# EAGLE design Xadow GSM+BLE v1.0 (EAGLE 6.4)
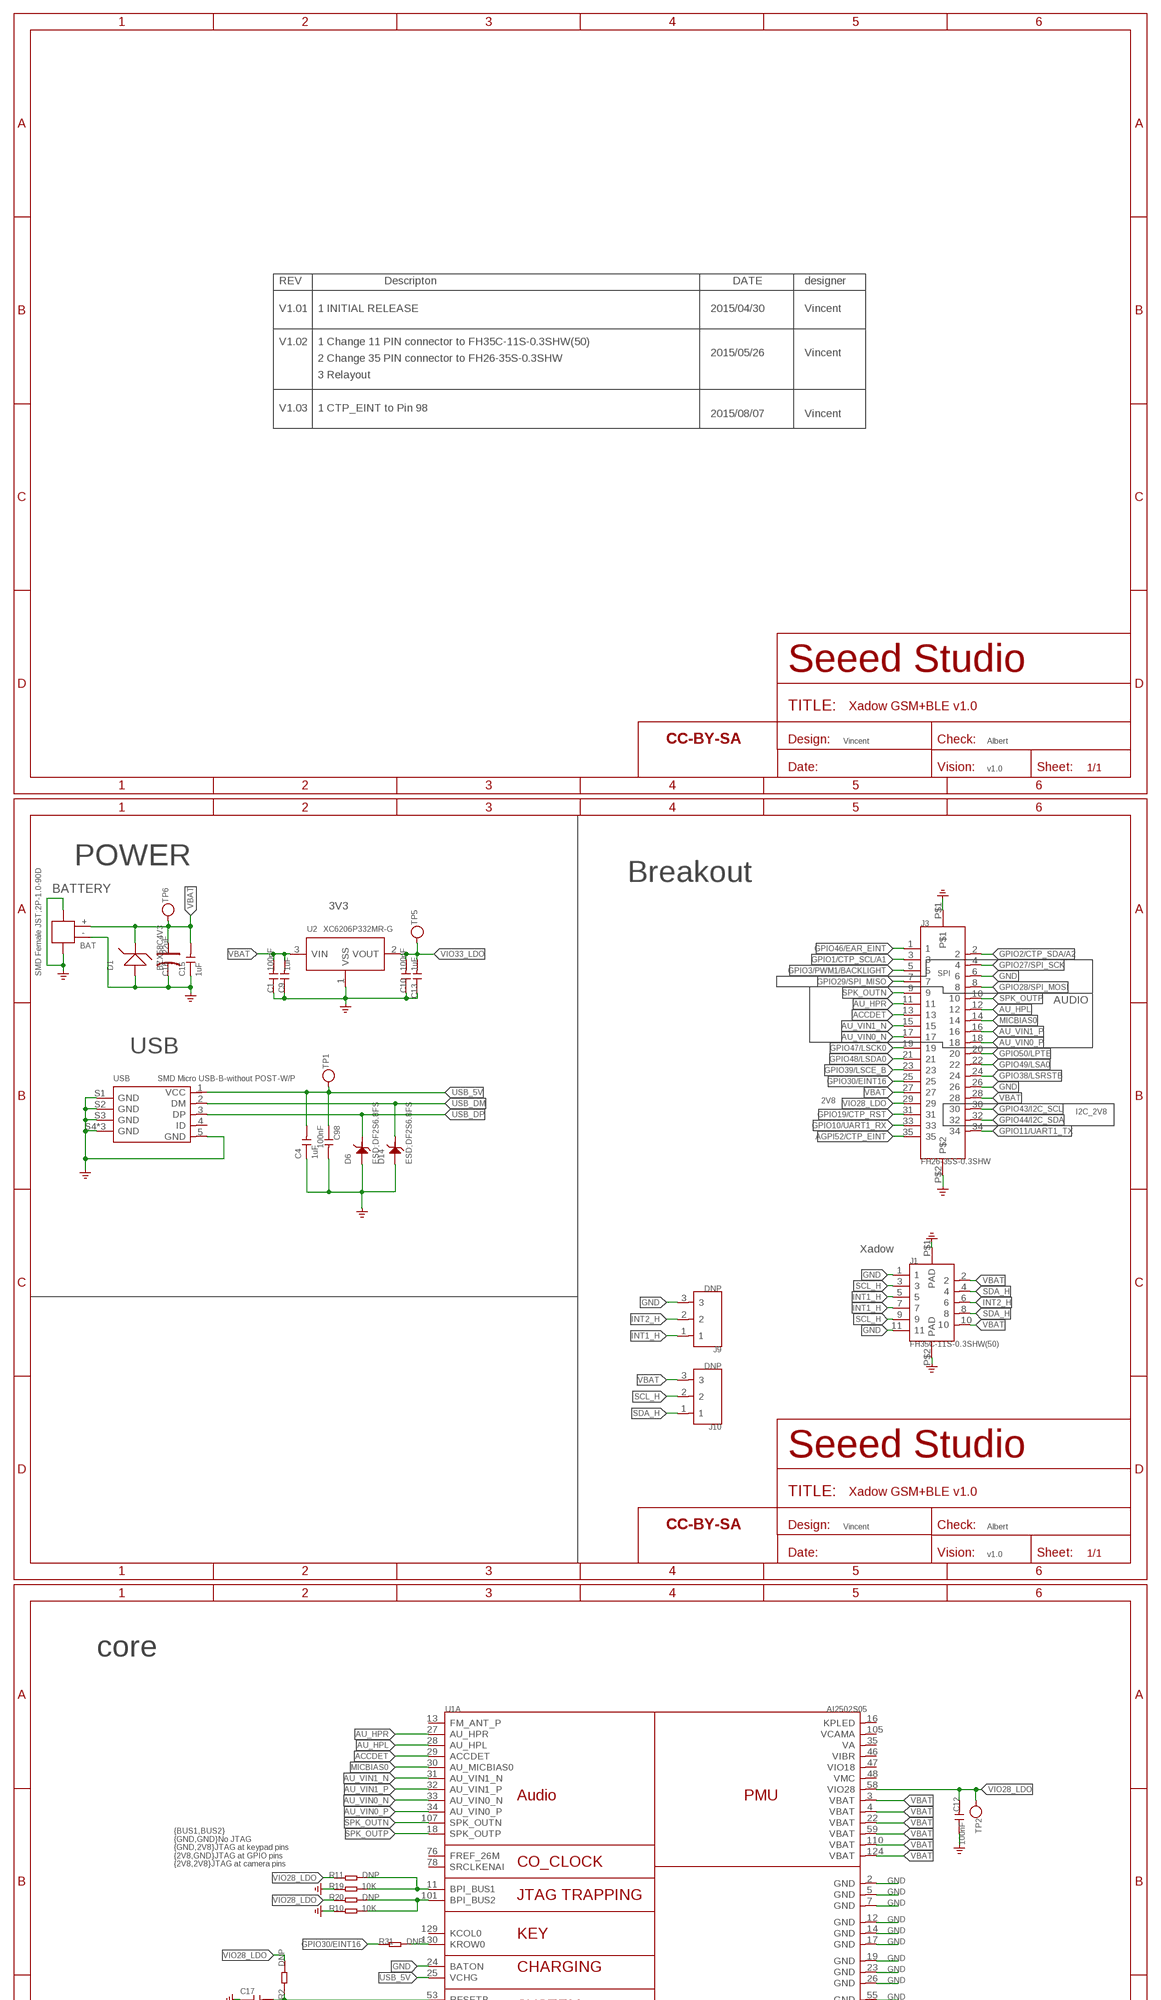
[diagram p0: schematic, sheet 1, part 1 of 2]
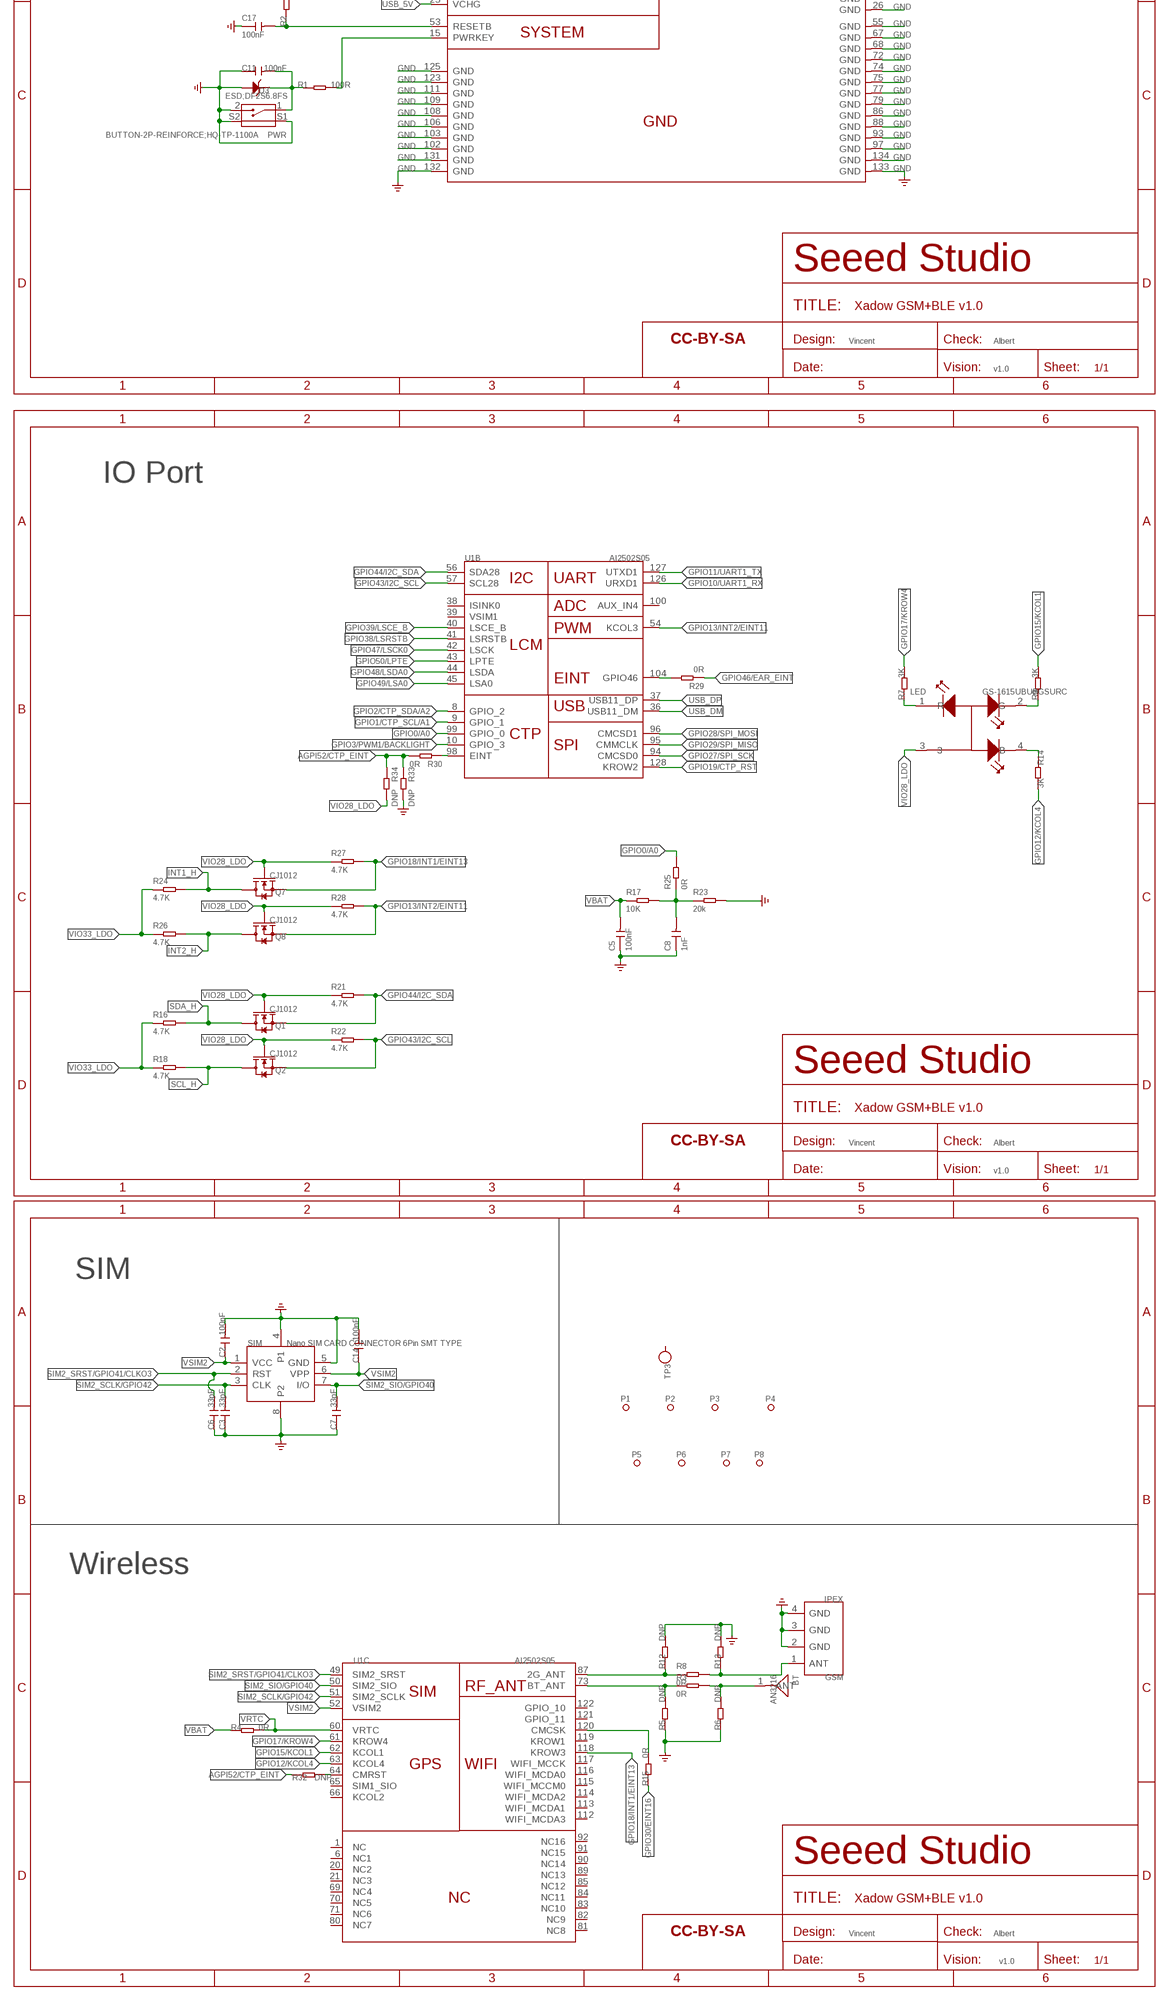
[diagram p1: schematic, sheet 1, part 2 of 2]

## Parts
BAT  SMD Female JST;2P-1.0-90D  JST-2P-SMD'1.0'  [HW2-SMD-1.0-90D]
BT  AN3216  ANTENNA-AN3216  [ANT-SMD2P-3.2X1.6X1.04MM]
C1  100nF  CAP-0201  [C0201]
C2  100nF  CAP-0201  [C0201]
C3  33pF  CAP-0201  [C0201]
C4  1uF  CAP-0402  [C0402]
C5  100nF  CAP-0201  [C0201]
C6  33pF  CAP-0201  [C0201]
C7  33pF  CAP-0201  [C0201]
C8  1nF  CAP-0201  [C0201]
C9  1uF  CAP-0402  [C0402]
C10  100nF  CAP-0201  [C0201]
C11  100nF  CAP-0201  [C0201]
C12  100nF  CAP-0201  [C0201]
C13  1uF  CAP-0402  [C0402]
C14  100nF  CAP-0201  [C0201]
C15  1uF  CAP-0402  [C0402]
C16  22uF  CAP-POLAR-AVX-A  [AVX-A]
C17  100nF  CAP-0201  [C0201]
C98  100nF  CAP-0201  [C0201]
D1  BZX58C4V3  D-ZENER-2P'BZX584CX'  [SOD-523]
D3  ESD;DF2S6.8FS  D-ESD-2P'DF2S6.8FS'  [SOD-923]
D6  ESD;DF2S6.8FS  D-ESD-2P'DF2S6.8FS'  [SOD-923]
D14  ESD;DF2S6.8FS  D-ESD-2P'DF2S6.8FS'  [SOD-923]
FR1  SEEEDSTUDIO-OPEN-SCH-FRAME  [SEEEDSTUDIO-PCB-FRAME]
GSM  IPEX  ANT_IPEX  [ANT-IPEX4-1.7X1.7MM]
J1  FH35C-11S-0.3SHW(50)  FPC-CONNECTER-11P(FH35C-11S-0.3SHW(50))  [FPC11-SMD-0.3(FH35C)]
J3  FH26-35S-0.3SHW  FPC-CONNECTER-35P(FH26W-35S-0.3SHW(10))  [FPC35-SMD-0.3(FH26W)]
J9  DNP  HEADER3  [3P-DIP-2]
J10  DNP  HEADER3  [3P-DIP-2]
LED  GS-1615UBUBGSURC  LED-GS-0603RGB  [LED-SMD4P-1.6X1.5MM]
P1  MARK-1.0'ANNULAR'  [ROUND-MARK-1.0]
P2  MARK-1.0'ANNULAR'  [ROUND-MARK-1.0]
P3  MARK-1.0'ANNULAR'  [ROUND-MARK-1.0]
P4  MARK-1.0'ANNULAR'  [ROUND-MARK-1.0]
P5  MARK-1.0'ANNULAR'  [ROUND-MARK-1.0]
P6  MARK-1.0'ANNULAR'  [ROUND-MARK-1.0]
P7  MARK-1.0'ANNULAR'  [ROUND-MARK-1.0]
P8  MARK-1.0'ANNULAR'  [ROUND-MARK-1.0]
PWR  BUTTON-2P-REINFORCE;HQ-TP-1100A  BUTTON-2+2P'HQ-TP-1100A'  [SW4-SMD-4.5X3.8X1.8MM-90D]
Q1  CJ1012  MOSFET-N  [SOT-523]
Q2  CJ1012  MOSFET-N  [SOT-523]
Q7  CJ1012  MOSFET-N  [SOT-523]
Q8  CJ1012  MOSFET-N  [SOT-523]
R1  100R  RES-0201  [R0201]
R2  DNP  RES-0201  [R0201]
R3  0R  RES-0201  [R0201]
R4  0R  RES-0201  [R0201]
R5  DNP  RES-0201  [R0201]
R6  DNP  RES-0201  [R0201]
R7  3K  RES-0201  [R0201]
R8  0R  RES-0201  [R0201]
R9  3K  RES-0201  [R0201]
R10  10K  RES-0201  [R0201]
R11  DNP  RES-0201  [R0201]
R12  DNP  RES-0201  [R0201]
R13  DNP  RES-0201  [R0201]
R14  3K  RES-0201  [R0201]
R15  0R  RES-0201  [R0201]
R16  4.7K  RES-0201  [R0201]
R17  10K  RES-0201  [R0201]
R18  4.7K  RES-0201  [R0201]
R19  10K  RES-0201  [R0201]
R20  DNP  RES-0201  [R0201]
R21  4.7K  RES-0201  [R0201]
R22  4.7K  RES-0201  [R0201]
R23  20k  RES-0201  [R0201]
R24  4.7K  RES-0201  [R0201]
R25  0R  RES-0201  [R0201]
R26  4.7K  RES-0201  [R0201]
R27  4.7K  RES-0201  [R0201]
R28  4.7K  RES-0201  [R0201]
R29  0R  RES-0201  [R0201]
R30  0R  RES-0201  [R0201]
R31  DNP  RES-0201  [R0201]
R32  DNP  RES-0201  [R0201]
R33  DNP  RES-0201  [R0201]
R34  DNP  RES-0201  [R0201]
SIM  Nano SIM CARD CONNECTOR 6Pin SMT TYPE  NANO-SIM-6+2P-SMD  [NANO-SIM6+2P-SMD-12.3X10X1.5MM]
TP1  PAD-TEST-POINT  [TP-D23MIL]
TP2  PAD-TEST-POINT  [TP-D23MIL]
TP3  PAD-TEST-POINT  [TP-D23MIL]
TP5  PAD-TEST-POINT  [TP-D23MIL]
TP6  PAD-TEST-POINT  [TP-D23MIL]
U1  AI2502S05  MODULE-MT2502A  [LGA134-0.6-17X15MM]
U2  XC6206P332MR-G  PMIC-XC6206PMR  [SOT-23]
U$1  SEEEDSTUDIO-OPEN-SCH-FRAME  [SEEEDSTUDIO-PCB-FRAME]
U$3  SEEEDSTUDIO-OPEN-SCH-FRAME  [SEEEDSTUDIO-PCB-FRAME]
U$5  SEEEDSTUDIO-OPEN-SCH-FRAME  [SEEEDSTUDIO-PCB-FRAME]
U$11  SEEEDSTUDIO-OPEN-SCH-FRAME  [SEEEDSTUDIO-PCB-FRAME]
USB  SMD Micro USB-B-without POST-W/P  MICRO-USB5+4P  [MICRO-USB5+4P-SMD-0.65-B-NO-HOLE]

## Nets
ACCDET: J3.13 U1.29(A:ACCDET)
AGPI52/CTP_EINT: J3.35 R30.2 R32.1 R33.1 R34.1
AU_HPL: J3.12 U1.28(A:AU_HPL)
AU_HPR: J3.11 U1.27(A:AU_HPR)
AU_VIN0_N: J3.17 U1.33(A:AU_VIN0_N)
AU_VIN0_P: J3.18 U1.34(A:AU_VIN0_P)
AU_VIN1_N: J3.15 U1.31(A:AU_VIN1_N)
AU_VIN1_P: J3.16 U1.32(A:AU_VIN1_P)
GND: BAT.3 BAT.4 BAT.- C1.1 C2.2 C3.1 C4.1 C5.1 C6.1 C7.1 C8.1 C9.1 C10.1 C11.1 C12.1 C13.1 C14.2 C15.1 C16.- C17.1 C98.2 D1.+ D3.2 D6.2 D14.2 GSM.2(GND) GSM.3(GND) GSM.4(GND) J1.1 J1.11 J1.P$1(PAD) J1.P$2(PAD) J3.6 J3.26 J3.P$1 J3.P$2 J9.3 PWR.2 PWR.S1 PWR.S2 R5.1 R6.1 R10.1 R12.2 R13.2 R19.1 R23.2 R33.2 SIM.4(P1) SIM.5(GND) SIM.8(P2) U1.2(A:GND) U1.5(A:GND) U1.7(A:GND) U1.12(A:GND) U1.14(A:GND) U1.17(A:GND) U1.19(A:GND) U1.23(A:GND) U1.24(A:BATON) U1.26(A:GND) U1.55(A:GND) U1.67(A:GND) U1.68(A:GND) U1.72(A:GND) U1.74(A:GND) U1.75(A:GND) U1.77(A:GND) U1.79(A:GND) U1.86(A:GND) U1.88(A:GND) U1.93(A:GND) U1.97(A:GND) U1.102(A:GND) U1.103(A:GND) U1.106(A:GND) U1.108(A:GND) U1.109(A:GND) U1.111(A:GND) U1.123(A:GND) U1.125(A:GND) U1.131(A:GND) U1.132(A:GND) U1.133(A:GND) U1.134(A:GND) U2.1(VSS) USB.5(GND) USB.S1(GND) USB.S2(GND) USB.S3(GND) USB.S4(GND) USB.S5(GND) USB.S6(GND) ; supply symbol labelled GND_POWER
GPIO0/A0: R25.2 U1.99(B:GPIO_0)
GPIO1/CTP_SCL/A1: J3.3 U1.9(B:GPIO_1)
GPIO2/CTP_SDA/A2: J3.2 U1.8(B:GPIO_2)
GPIO3/PWM1/BACKLIGHT: J3.5 U1.10(B:GPIO_3)
GPIO10/UART1_RX: J3.33 U1.126(B:URXD1)
GPIO11/UART1_TX: J3.34 U1.127(B:UTXD1)
GPIO12/KCOL4: R14.2 U1.63(C:KCOL4)
GPIO13/INT2/EINT11: Q8.2(S) R28.2 U1.54(B:KCOL3)
GPIO15/KCOL1: R9.2 U1.62(C:KCOL1)
GPIO17/KROW4: R7.2 U1.61(C:KROW4)
GPIO18/INT1/EINT13: Q7.2(S) R27.2 U1.118(C:KROW3)
GPIO19/CTP_RST: J3.31 U1.128(B:KROW2)
GPIO27/SPI_SCK: J3.4 U1.94(B:CMCSD0)
GPIO28/SPI_MOSI: J3.8 U1.96(B:CMCSD1)
GPIO29/SPI_MISO: J3.7 U1.95(B:CMMCLK)
GPIO30/EINT16: J3.25 R15.1 R31.1
GPIO38/LSRSTB: J3.24 U1.41(B:LSRSTB)
GPIO39/LSCE_B: J3.23 U1.40(B:LSCE_B)
GPIO43/I2C_SCL: J3.30 Q2.2(S) R22.2 U1.57(B:SCL28)
GPIO44/I2C_SDA: J3.32 Q1.2(S) R21.2 U1.56(B:SDA28)
GPIO46/EAR_EINT: J3.1 R29.1
GPIO47/LSCK0: J3.19 U1.42(B:LSCK)
GPIO48/LSDA0: J3.21 U1.44(B:LSDA)
GPIO49/LSA0: J3.22 U1.45(B:LSA0)
GPIO50/LPTE: J3.20 U1.43(B:LPTE)
INT1_H: J1.5 J1.7 J9.1 Q7.3(D) R24.2
INT2_H: J1.6 J9.2 Q8.3(D) R26.2
MICBIAS0: J3.14 U1.30(A:AU_MICBIAS0)
N$1: R15.2 U1.120(C:CMCSK)
N$2: R29.2 U1.104(B:GPIO46)
N$3: R30.1 U1.98(B:EINT)
N$4: BT.1(ANT) R3.2 R6.2
N$5: R8.1 R12.1 U1.87(C:2G_ANT)
N$6: R31.2 U1.130(A:KROW0)
N$7: GSM.1(ANT) R8.2 R13.1
N$8: C11.2 D3.1 PWR.1 R1.1
N$9: R3.1 R5.2 U1.73(C:BT_ANT)
N$10: R1.2 U1.15(A:PWRKEY)
N$12: C8.2 R17.2 R23.1 R25.1
N$18: R32.2 U1.64(C:CMRST)
N$20: R10.2 R20.2 U1.101(A:BPI_BUS2)
N$21: R11.2 R19.2 U1.11(A:BPI_BUS1)
N$32: LED.1(R) R7.1
N$33: LED.2(G) R9.1
N$34: LED.4(B) R14.1
RESETB: C17.2 R2.1 U1.53(A:RESETB)
SCL_H: J1.3 J1.9 J10.2 Q2.3(D) R18.2
SDA_H: J1.4 J1.8 J10.1 Q1.3(D) R16.2
SIM2_SCLK/GPIO42: C3.2 SIM.3(CLK) U1.51(C:SIM2_SCLK)
SIM2_SIO/GPIO40: C7.2 SIM.7(I/O) U1.50(C:SIM2_SIO)
SIM2_SRST/GPIO41/CLKO3: C6.2 SIM.2(RST) U1.49(C:SIM2_SRST)
SPK_OUTN: J3.9 U1.107(A:SPK_OUTN)
SPK_OUTP: J3.10 U1.18(A:SPK_OUTP)
USB_5V: C4.2 C98.1 TP1.T U1.25(A:VCHG) USB.1(VCC)
USB_DM: D14.1 U1.36(B:USB11_DM) USB.2(DM)
USB_DP: D6.1 U1.37(B:USB11_DP) USB.3(DP)
VBAT: BAT.+ C1.2 C5.2 C9.2 C15.2 C16.+ D1.- J1.2 J1.10 J3.27 J3.28 J10.3 R4.1 R17.1 TP6.T U1.3(A:VBAT) U1.4(A:VBAT) U1.22(A:VBAT) U1.59(A:VBAT) U1.110(A:VBAT) U1.124(A:VBAT) U2.3(VIN)
VIO28_LDO: C12.2 J3.29 LED.3 Q1.1(G) Q2.1(G) Q7.1(G) Q8.1(G) R2.2 R11.1 R20.1 R21.1 R22.1 R27.1 R28.1 R34.2 TP2.T U1.58(A:VIO28)
VIO33_LDO: C10.2 C13.2 R16.1 R18.1 R24.1 R26.1 TP5.T U2.2(VOUT)
VRTC: R4.2 U1.60(C:VRTC)
VSIM2: C2.1 C14.1 SIM.1(VCC) SIM.6(VPP) U1.52(C:VSIM2)
Unconnected: TP3.T U1.1(C:NC) U1.6(C:NC1) U1.13(A:FM_ANT_P) U1.16(A:KPLED) U1.20(C:NC2) U1.21(C:NC3) U1.35(A:VA) U1.38(B:ISINK0) U1.39(B:VSIM1) U1.46(A:VIBR) U1.47(A:VIO18) U1.48(A:VMC) U1.65(C:SIM1_SIO) U1.66(C:KCOL2) U1.69(C:NC4) U1.70(C:NC5) U1.71(C:NC6) U1.76(A:FREF_26M) U1.78(A:SRCLKENAI) U1.80(C:NC7) U1.81(C:NC8) U1.82(C:NC9) U1.83(C:NC10) U1.84(C:NC11) U1.85(C:NC12) U1.89(C:NC13) U1.90(C:NC14) U1.91(C:NC15) U1.92(C:NC16) U1.100(B:AUX_IN4) U1.105(A:VCAMA) U1.112(C:WIFI_MCDA3) U1.113(C:WIFI_MCDA1) U1.114(C:WIFI_MCDA2) U1.115(C:WIFI_MCCM0) U1.116(C:WIFI_MCDA0) U1.117(C:WIFI_MCCK) U1.119(C:KROW1) U1.121(C:GPIO_11) U1.122(C:GPIO_10) U1.129(A:KCOL0) USB.4(ID)

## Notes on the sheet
- REV | Descripton | DATE | designer
- V1.01 | 1 INITIAL RELEASE | 2015/04/30 | Vincent
- V1.02 | 1 Change 11 PIN connector to FH35C-11S-0.3SHW(50)
- 2015/05/26 | Vincent
- 2 Change 35 PIN connector to FH26-35S-0.3SHW
- 3 Relayout
- V1.03 | 1 CTP_EINT to Pin 98
- 2015/08/07 | Vincent
- Vincent | Albert
- v1.0
- POWER
- Breakout
- BATTERY
- 3V3
- SPI
- AUDIO
- USB
- 2V8
- I2C_2V8
- Xadow
- Vincent | Albert
- v1.0
- core
- {BUS1,BUS2}
- {GND,GND}No JTAG
  {GND,2V8}JTAG at keypad pins
  {2V8,GND}JTAG at GPIO pins
  {2V8,2V8}JTAG at camera pins
- Vincent | Albert
- v1.0
- IO Port
- Vincent | Albert
- v1.0
- SIM
- Wireless
- Vincent | Albert
- v1.0

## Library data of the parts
BAT = Connector-new:JST-2P-SMD: 2P-SMD-1.0-90D:320110054;2P-SMD-2.0-90D:320110026
BT = template:ANTENNA-AN3216
C1-C15 C17 C98 = Discrete-new:CAP: Ceramic Capacitors
C16 = Discrete-new:CAP-POLAR: Electrolytic Capacitors,Tantalum Capacitors and Super Capacitors
D1 = Discrete-new:D-ZENER-2P: SOD-123:304030008;SOT-23:304030000
D3 D6 D14 = Discrete-new:D-ESD-2P: SOD-923:304060009;SOD-123:304060001
FR1 U$1 U$3 U$5 U$11 = moudle-new:SEEEDSTUDIO-OPEN-SCH-FRAME
GSM = template:ANT_IPEX
J1 = template:FPC-CONNECTER-11P(FH35C-11S-0.3SHW(50))
J3 = template:FPC-CONNECTER-35P(FH26W-35S-0.3SHW(10))
J9 J10 = template:HEADER3
LED = template:LED-GS-0603RGB
P1-P8 = Discrete-new:MARK-1.0; PARTNO: DNP
PWR = Discrete-new:BUTTON-2+2P: SW4-SMD-4.5X3.8X1.8MM-90D:311020035;SW4-SMD-7.0X3.5X3.5MM-90D:311020023
Q1 Q2 Q7 Q8 = template:MOSFET-N: IRLL014: http://www.vishay.com/docs/91319/sihll014.pdf
R1-R34 = Discrete-new:RES
SIM = template:NANO-SIM-6+2P-SMD
TP1-TP3 TP5 TP6 = Discrete-new:PAD-TEST-POINT
U1 = moudle-new:MODULE-MT2502A
U2 = IC-new:PMIC-XC6206P: LOW ESR Cap.Compatible Positive Voltage Regulators
USB = Connector-new:MICRO-USB5+4P: 5+4P-SMD-0.65-B:320010000;5+2P-SMD-0.65-AB:340032001

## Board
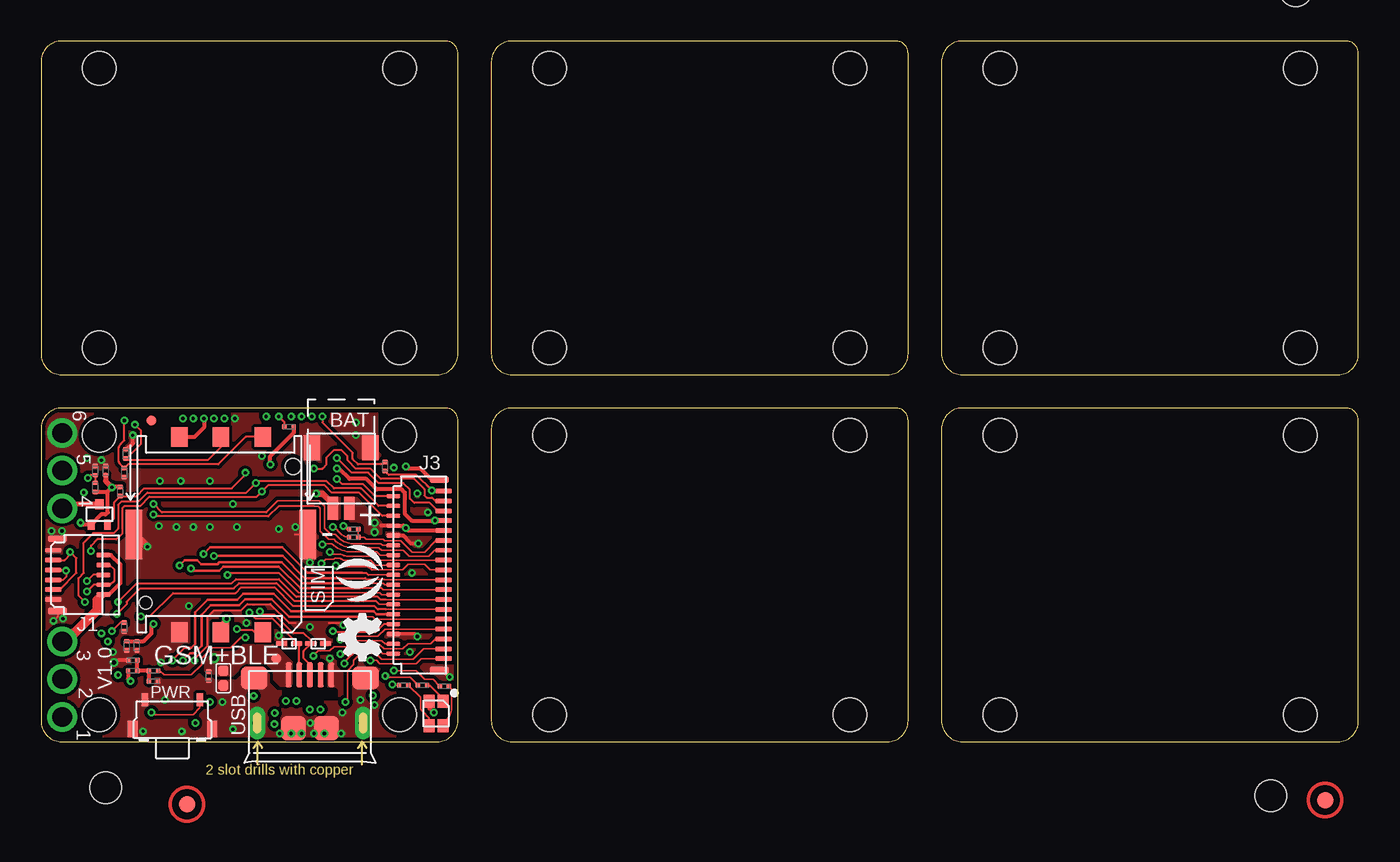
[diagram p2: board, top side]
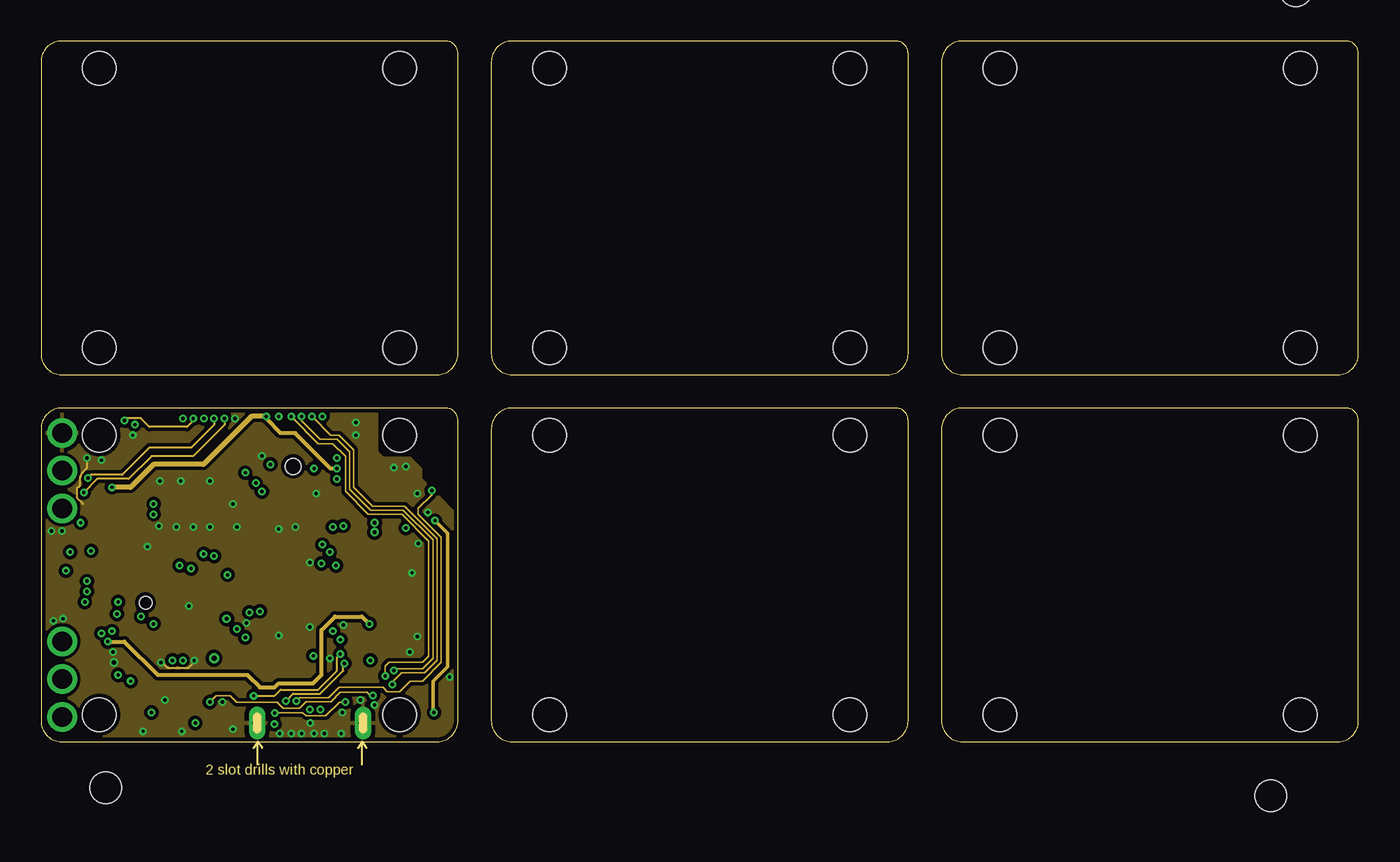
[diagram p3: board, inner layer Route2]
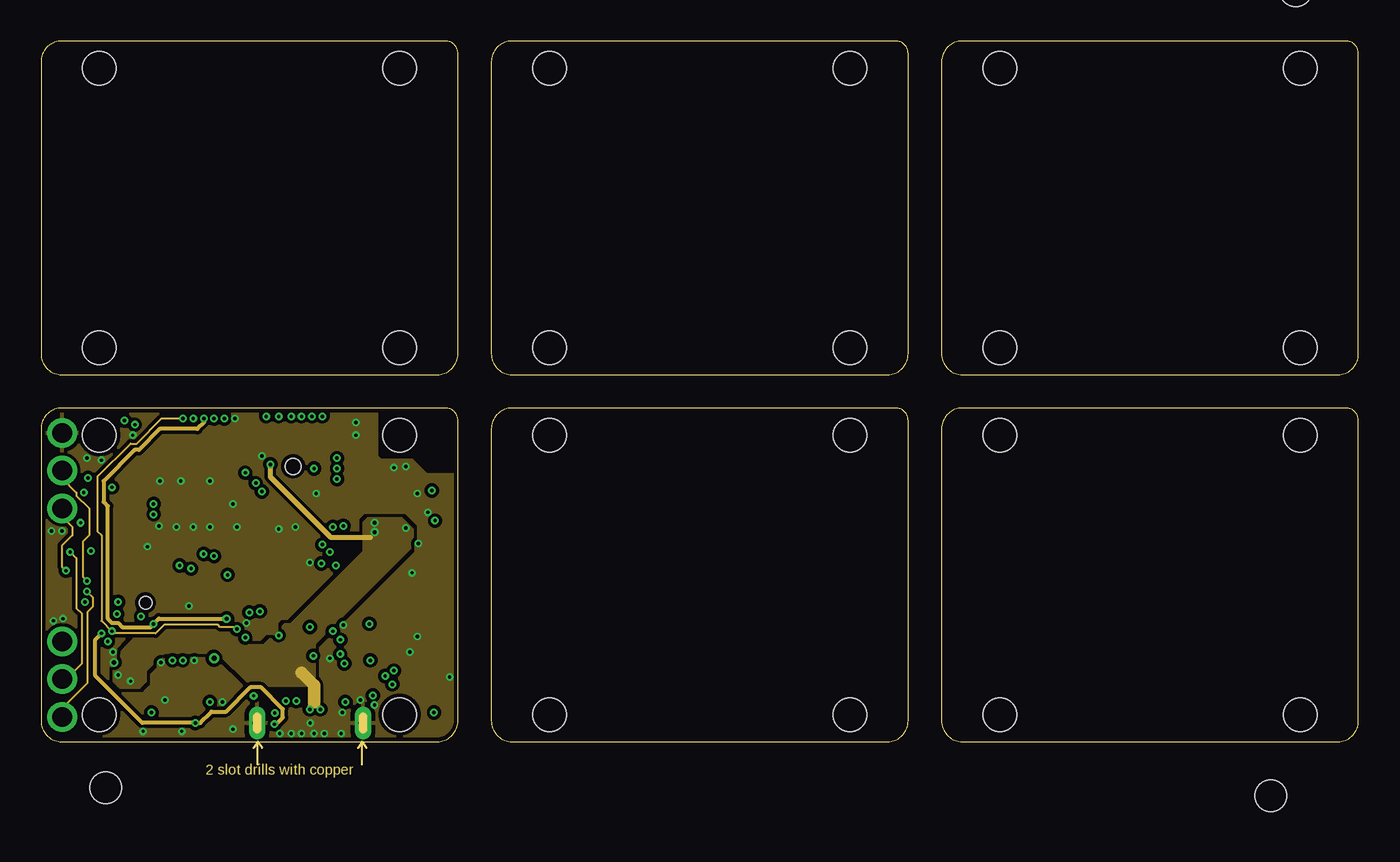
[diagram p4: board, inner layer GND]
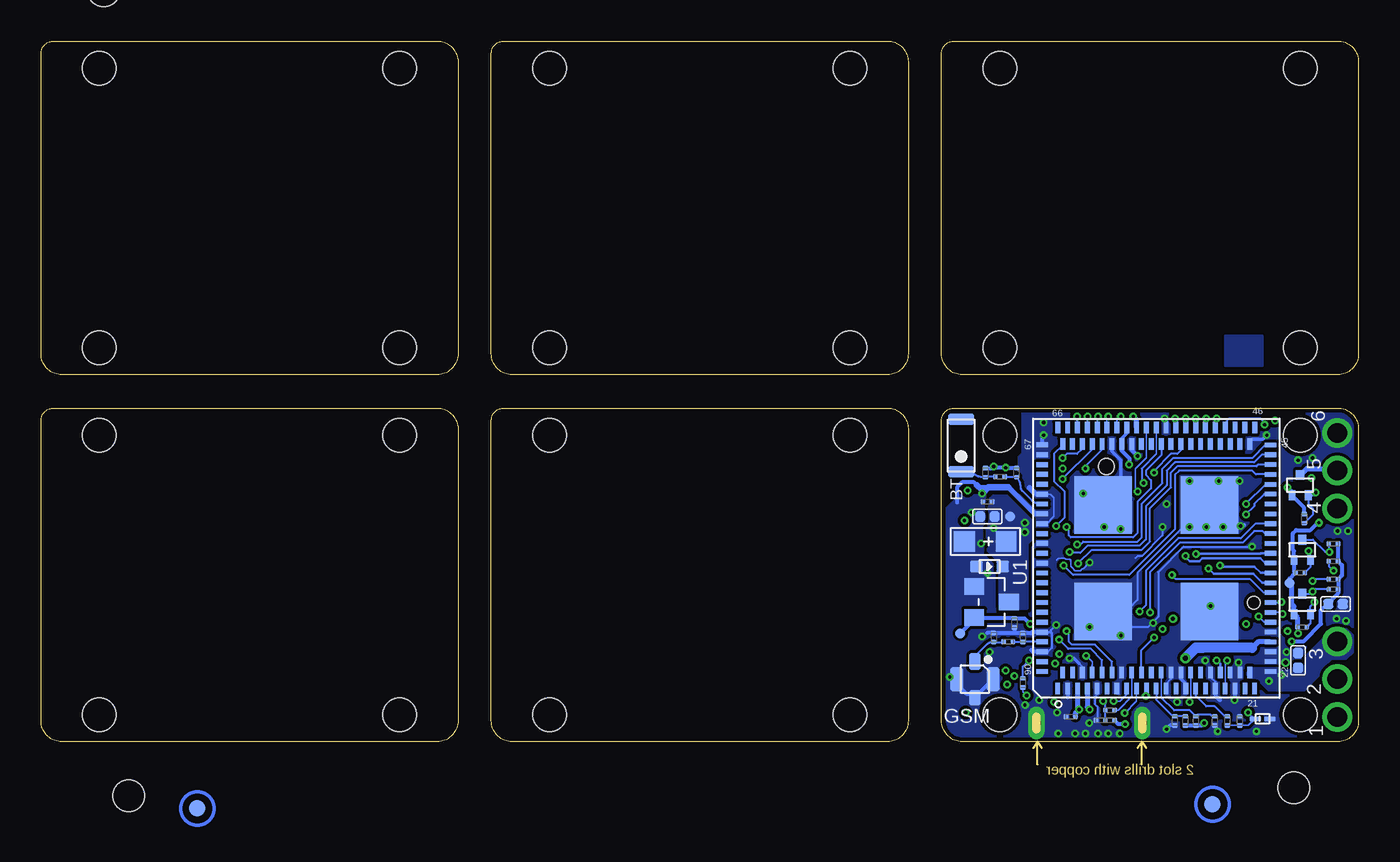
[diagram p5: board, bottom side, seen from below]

Size 80.26 x 42.67 mm. Coordinates in mm from the lower left corner, seen from the top.
Outline: 52 segments
Copper layers (1*2*15*16): Top 0.035mm / dielectric 0.2mm / Route2 0.0175mm / dielectric 0.3mm / GND 0.0175mm / dielectric 0.2mm / Bottom 0.035mm
Design rules "SeeedStudio_4layer_DRU_no_angle_20140221 *": minimum track width 0.09398125mm, minimum drill 8mil, track to track 5mil, track to pad 4mil, pad to pad 5mil, via to via 5mil, smd to smd 0mil, copper to edge 10mil, drill to drill 6mil, minimum pad ring 6mil, minimum via ring 4mil, stop-mask expansion 4mil, vias tented up to drill 100mil, thermal gap 10mil
Holes 2.03 mm at 3.56,1.65 3.56,18.67 21.84,18.67 21.84,1.65 3.56,24 3.56,41.02 21.84,41.02 21.84,24 30.99,1.65 30.99,18.67 49.28,18.67 49.28,1.65 30.99,24 30.99,41.02 49.28,41.02 49.28,24 58.42,1.65 58.42,18.67 76.71,18.67 76.71,1.65 58.42,24 58.42,41.02 76.71,41.02 76.71,24
Holes 1.91 mm at 3.94,-2.79 74.93,-3.3 76.45,45.72 3.17,46.61
tRestrict: area 21,15.2 to 25.4,20.3
bRestrict: area 21,15.2 to 25.4,20.3

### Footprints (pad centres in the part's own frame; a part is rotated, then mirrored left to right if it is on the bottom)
HW2-SMD-1.0-90D = smd 1.524 x 1.016: 3 -3.429,1.778; 4 -3.429,-1.778 | smd 1.397 x 0.635: + 0.254,0.508; - 0.254,-0.508
ANT-SMD2P-3.2X1.6X1.04MM = smd 1.6 x 0.7: 1 0,1.6; 2 0,-1.6
C0201 = smd 0.279 x 0.318: 1 -0.279,0; 2 0.279,0
C0402 = smd 0.635 x 0.635: 1 0,0.445; 2 0,-0.445
AVX-A = smd 1.27 x 1.27: + -1.27,0; - 1.27,0
SOD-523 = smd 0.762 x 0.7: + -0.8,0; - 0.8,0
SOD-923 = smd 0.7 x 0.3: 1 -0.45,0; 2 0.45,0
ANT-IPEX4-1.7X1.7MM = smd 0.7 x 1.05: 1 0,-1.075 | smd 0.8 x 1.5: 2 1.1,0; 4 -1.1,0 | smd 0.7 x 0.95: 3 0,1.125
FPC11-SMD-0.3(FH35C) = smd 0.3 x 1: 1 -1.5,-3.075; 3 -0.9,-3.075; 5 -0.3,-3.075; 7 0.3,-3.075; 9 0.9,-3.075; 11 1.5,-3.075 | smd 0.3 x 0.85: 2 -1.2,0; 4 -0.6,0; 6 0,0; 8 0.6,0; 10 1.2,0 | smd 0.4 x 1.15: P$1 2.2,-2.8; P$2 -2.2,-2.8
FPC35-SMD-0.3(FH26W) = smd 0.3 x 1: 1 -5.1,-1.551; 3 -4.5,-1.551; 5 -3.9,-1.551; 7 -3.3,-1.551; 9 -2.7,-1.551; 11 -2.1,-1.551; 13 -1.5,-1.551; 15 -0.9,-1.551; 17 -0.3,-1.551; 19 0.3,-1.551; 21 0.9,-1.551; 23 1.5,-1.551; 25 2.1,-1.551; 27 2.7,-1.551; 29 3.3,-1.551; 31 3.9,-1.551; 33 4.5,-1.551; 35 5.1,-1.551 | smd 0.254 x 0.851: 2 -4.8,1.524; 4 -4.2,1.524; 6 -3.6,1.524; 8 -3,1.524; 10 -2.4,1.524; 12 -1.8,1.524; 14 -1.2,1.524; 16 -0.6,1.524; 18 0,1.524; 20 0.6,1.524; 22 1.2,1.524; 24 1.8,1.524; 26 2.4,1.524; 28 3,1.524; 30 3.6,1.524; 32 4.2,1.524; 34 4.8,1.524 | smd 0.4 x 1.15: P$1 5.8,-1.276; P$2 -5.8,-1.276
3P-DIP-2 = drill 1.2 pad 1.8: 1 -2.3,-0.02; 2 0,-0.02; 3 2.3,-0.02
LED-SMD4P-1.6X1.5MM = smd 0.8 x 0.65: 1 -0.75,0.425; 2 0.75,0.425; 3 -0.75,-0.425; 4 0.75,-0.425
ROUND-MARK-1.0 = smd 1.016 x 1.016: P$1 0,0
SW4-SMD-4.5X3.8X1.8MM-90D = smd 0.4 x 0.8: 1 -1.675,-1.277; 2 1.675,-1.277 | smd 0.6 x 1: S1 -2.425,0.5; S2 2.425,0.5
SOT-523 = smd 0.4 x 0.6: 1 0.5,0.62; 2 -0.5,0.62 | smd 0.5 x 0.6: 3 0,-0.62
R0201 = smd 0.279 x 0.318: 1 -0.279,0; 2 0.279,0
NANO-SIM6+2P-SMD-12.3X10X1.5MM = smd 1 x 1.2: 1 6.94,-1.8; 2 4.4,-1.8; 3 1.86,-1.8; 5 6.94,10.1; 6 4.4,10.1; 7 1.86,10.1 | smd 1 x 3: 4 9.71,4.15; 8 -0.9,4.15 | hole 0.95: 0,0 | hole 0.75: 9,8.3
TP-D23MIL = smd 0.6 x 0.6: T 0,0
LGA134-0.6-17X15MM = smd 0.7 x 0.28: 1 -7.95,6; 2 -7.95,5.4; 3 -7.95,4.8; 4 -7.95,4.2; 5 -7.95,3.6; 6 -7.95,3; 7 -7.95,2.4; 8 -7.95,1.8; 9 -7.95,1.2; 10 -7.95,0.6; 11 -7.95,0; 12 -7.95,-0.6; 13 -7.95,-1.2; 14 -7.95,-1.8; 15 -7.95,-2.4; 16 -7.95,-3; 17 -7.95,-3.6; 18 -7.95,-4.2; 19 -7.95,-4.8; 20 -7.95,-5.4; 21 -7.95,-6; 91 -6.95,5.7; 92 -6.95,5.1; 93 -6.95,4.5; 94 -6.95,3.9; 95 -6.95,3.3; 96 -6.95,2.7; 97 -6.95,2.1; 98 -6.95,1.5; 99 -6.95,0.9; 100 -6.95,0.3; 101 -6.95,-0.3; 102 -6.95,-0.9; 103 -6.95,-1.5; 104 -6.95,-2.1; 105 -6.95,-2.7; 106 -6.95,-3.3; 107 -6.95,-3.9; 108 -6.95,-4.5; 109 -6.95,-5.1; 110 -6.95,-5.7 | smd 0.28 x 0.7: 22 -6.9,-6.95; 23 -6.3,-6.95; 24 -5.7,-6.95; 25 -5.1,-6.95; 26 -4.5,-6.95; 27 -3.9,-6.95; 28 -3.3,-6.95; 29 -2.7,-6.95; 30 -2.1,-6.95; 31 -1.5,-6.95; 32 -0.9,-6.95; 33 -0.3,-6.95; 34 0.3,-6.95; 35 0.9,-6.95; 36 1.5,-6.95; 37 2.1,-6.95; 38 2.7,-6.95; 39 3.3,-6.95; 40 3.9,-6.95; 41 4.5,-6.95; 42 5.1,-6.95; 43 5.7,-6.95; 44 6.3,-6.95; 45 6.9,-6.95 | smd 0.7 x 0.3: 46 7.95,-6; 47 7.95,-5.4; 48 7.95,-4.8; 49 7.95,-4.2; 50 7.95,-3.6; 51 7.95,-3; 52 7.95,-2.4; 53 7.95,-1.8; 54 7.95,-1.2; 55 7.95,-0.6; 56 7.95,0; 57 7.95,0.6; 58 7.95,1.2; 59 7.95,1.8; 60 7.95,2.4; 61 7.95,3; 62 7.95,3.6; 63 7.95,4.2; 64 7.95,4.8; 65 7.95,5.4; 66 7.95,6; 111 6.95,-5.7; 112 6.95,-5.1; 113 6.95,-4.5; 114 6.95,-3.9; 115 6.95,-3.3; 116 6.95,-2.7; 117 6.95,-2.1; 118 6.95,-1.5; 119 6.95,-0.9; 120 6.95,-0.3; 121 6.95,0.3; 122 6.95,0.9; 123 6.95,1.5; 124 6.95,2.1; 125 6.95,2.7; 126 6.95,3.3; 127 6.95,3.9; 128 6.95,4.5; 129 6.95,5.1; 130 6.95,5.7 | smd 0.3 x 0.7: 67 6.9,6.95; 68 6.3,6.95; 69 5.7,6.95; 70 5.1,6.95; 71 4.5,6.95; 72 3.9,6.95; 73 3.3,6.95; 74 2.7,6.95; 75 2.1,6.95; 76 1.5,6.95; 77 0.9,6.95; 78 0.3,6.95; 79 -0.3,6.95; 80 -0.9,6.95; 81 -1.5,6.95; 82 -2.1,6.95; 83 -2.7,6.95; 84 -3.3,6.95; 85 -3.9,6.95; 86 -4.5,6.95; 87 -5.1,6.95; 88 -5.7,6.95; 89 -6.3,6.95; 90 -6.9,6.95 | smd 3.5 x 3.5: 131 3.25,3.25; 132 -3.25,3.25; 133 -3.25,-3.25; 134 3.25,-3.25
SOT-23 = smd 1.016 x 1.2: 1 -0.95,-1.06; 2 0.95,-1.06; 3 0,1.06
MICRO-USB5+4P-SMD-0.65-B-NO-HOLE = smd 0.381 x 1.524: 1 -1.3,-0.25; 2 -0.65,-0.25; 3 0,-0.25; 4 0.65,-0.25; 5 1.3,-0.25 | smd 1.6 x 1.397: S1 -3.4,-0.427; S6 3.4,-0.427 | drill 0.508 pad 1.016 long: S2 -3.226,-3.175; S5 3.226,-3.175 | smd 1.5 x 1.5: S3 -1,-3.5; S4 1,-3.5

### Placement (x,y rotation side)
BAT  18.29,14.48 270 top
BT  24.21,18.03 180 bottom
C1  22.61,14.61 0 bottom
C2  5.21,5.84 270 top
C3  5.08,16.38 90 top
C4  11.11,3.87 180 top
C5  17.53,1.52 0 bottom
C6  5.14,17.53 270 top
C7  5.08,6.99 90 top
C8  5.59,4.95 0 top
C9  3.68,4.95 0 bottom
C10  20.95,7.24 90 bottom
C11  7.24,1.27 270 bottom
C12  3.94,16.51 270 top
C13  1.4,8.38 270 bottom
C14  5.84,5.84 270 top
C15  22.61,13.72 90 bottom
C16  22.73,12.19 180 bottom
C17  3.3,16.51 270 top
C98  10.22,4 270 top
D1  22.48,10.67 0 bottom
D3  5.84,1.4 0 bottom
D6  16.89,5.97 0 top
D14  15.11,5.97 180 top
FR1  not placed on the board
GSM  23.37,3.81 180 bottom
J1  3.81,10.16 270 top
J3  22.99,10.16 90 top
J9  1.27,16.51 90 top
J10  1.27,3.81 90 top
LED  24.07,1.71 270 top
P1  not placed on the board
P2  not placed on the board
P3  not placed on the board
P4  not placed on the board
P5  not placed on the board
P6  not placed on the board
P7  not placed on the board
P8  not placed on the board
PWR  8,1.27 180 top
Q1  3.43,8.38 180 bottom
Q2  3.43,11.68 180 bottom
Q7  3.56,13.84 180 top
Q8  3.56,15.62 180 bottom
R1  8,1.27 90 bottom
R2  3.3,15.49 270 top
R3  21.84,16.13 180 bottom
R4  15.11,19.18 180 top
R5  20.83,16.38 270 bottom
R6  22.73,16.38 270 bottom
R7  23.24,3.43 180 top
R8  21.34,6.1 180 bottom
R9  24.57,3.37 180 top
R10  8.76,1.27 90 bottom
R11  10.54,1.27 90 bottom
R12  20.45,6.35 90 bottom
R13  22.23,6.35 90 bottom
R14  22.1,3.43 180 top
R15  19.05,12.45 180 top
R16  1.52,9.27 180 bottom
R17  5.59,4.32 0 top
R18  1.52,12.06 180 bottom
R19  11.18,1.27 90 bottom
R20  9.91,1.27 90 bottom
R21  3.43,6.99 0 bottom
R22  3.56,10.29 0 bottom
R23  6.86,3.68 0 top
R24  1.52,10.99 180 bottom
R25  6.86,4.32 0 top
R26  1.52,9.91 180 bottom
R27  4.83,15.24 270 top
R28  3.3,13.59 270 bottom
R29  20.45,3.58 270 bottom
R30  15.14,1.93 180 bottom
R31  19.05,12.95 180 top
R32  20.95,16.76 90 top
R33  15.7,1.3 180 bottom
R34  15.14,1.3 0 bottom
SIM  15.37,16.76 180 top
TP1  14.35,5.08 0 top
TP2  4.19,9.65 180 bottom
TP3  6.73,19.56 0 top
TP5  24.26,6.6 0 bottom
TP6  21.21,13.72 0 bottom
U1  12.32,11.18 90 bottom
U2  22.35,8.51 270 bottom
U$1  not placed on the board
U$2  [SEEED-SILK-160*153MIL]  19.3,10.29 90 top
U$3  not placed on the board
U$5  not placed on the board
U$11  not placed on the board
U$14  [OSHW_FILLX100_NOTEXT]  20.7,4.95 90 top
USB  16.38,4.32 0 top

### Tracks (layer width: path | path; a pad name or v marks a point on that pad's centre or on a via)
ACCDET  (via drill 0.2 pad 0.46)
  Top 0.094: J3.13 20.99,8.66
  Top 0.127: v4.7,8.51 5.84,9.65 11.62,9.65 11.87,9.91 14.48,9.91 15.56,8.83 20.51,8.83 20.68,8.66 20.99,8.66
  Bottom 0.102: U1.29 4.73,8.48 v4.7,8.51
AGPI52/CTP_EINT  (via drill 0.2 pad 0.46)
  Top 0.127: R32.1 21.18,16.26 22.86,16.26 v23.81,15.3 | J3.35 23.86,15.26 v23.81,15.3 | 23.49,15.62 v23.81,15.3
  Route2 0.102: v23.81,15.3 23.81,15.05 22.99,14.22 22.99,13.84 24.38,12.45 24.38,4.83 23.24,3.68 22.48,3.68 21.84,3.05 21.08,3.05 20.83,3.3 18.16,3.3 17.53,2.67 15.75,2.67 v15.56,2.48
  Bottom 0.127: R34.1 R30.2 15.42,2.34 v15.56,2.48
AU_HPL  (via drill 0.2 pad 0.46)
  Top 0.102: J3.12 20.6,8.36 20.38,8.57
  Top 0.127: v4.62,7.77 5.21,8.36 5.21,8.51 6.03,9.33 11.75,9.33 12.06,9.65 14.35,9.65 15.43,8.57 20.38,8.57
  Bottom 0.102: U1.28 4.73,7.88 v4.62,7.77
AU_HPR  (via drill 0.2 pad 0.46)
  Top 0.102: J3.11 21.02,8.06
  Top 0.127: v6.1,7.62 6.6,7.62 8.04,9.06 11.85,9.06 12.19,9.4 14.22,9.4 15.37,8.26 20.32,8.26 20.52,8.06 21.02,8.06
  Bottom 0.127: U1.27 5.75,7.28 v6.1,7.62
AU_VIN0_N  (via drill 0.2 pad 0.46)
  Top 0.094: 19.75,9.97 19.81,9.91 20.89,9.91 20.94,9.86 J3.17
  Top 0.127: 18.22,9.97 19.75,9.97
  Top 0.152: v10.54,11.3 10.56,11.33 14.71,11.33 16.06,9.97 18.22,9.97
  Bottom 0.152: U1.33 5.68,10.88 5.97,11.16 9.51,11.16 9.69,10.99 10.29,10.99 10.54,11.24 v10.54,11.3
AU_VIN0_P  (via drill 0.2 pad 0.46)
  Top 0.094: 19.94,10.16 21.02,10.16
  Top 0.102: J3.18 21.02,10.16
  Top 0.127: 19.56,10.29 19.81,10.29 19.94,10.16
  Top 0.152: v9.91,11.43 10.32,11.84 14.7,11.84 16.26,10.29 19.56,10.29
  Bottom 0.152: U1.34 5.94,11.48 5.97,11.44 9.89,11.44 v9.91,11.43
AU_VIN1_N  (via drill 0.2 pad 0.46)
  Top 0.094: 21.03,9.26 20.84,9.26 20.77,9.33
  Top 0.102: J3.15 21.03,9.26
  Top 0.127: 20.77,9.33 19.37,9.33
  Top 0.152: v9.14,10.54 9.27,10.41 10.86,10.41 11.1,10.65 14.49,10.65 15.81,9.33 19.37,9.33
  Bottom 0.152: U1.31 5.87,9.68 6.41,10.22 8.83,10.22 v9.14,10.54
AU_VIN1_P  (via drill 0.2 pad 0.46)
  Top 0.102: J3.16 20.92,9.56 20.83,9.65 19.49,9.65
  Top 0.152: 19.49,9.65 15.94,9.65 14.66,10.94 10.86,10.94 10.75,10.82 9.75,10.82 9.52,11.05 8.76,11.05 v8.45,10.73
  Bottom 0.152: U1.32 5.96,10.28 6.35,10.67 8.38,10.67 v8.45,10.73
GND  (via drill 0.2 pad 0.46, 0.25 pad 0.51)
  Top 0.127: SIM.8 15.45,12.61 | J1.P$1 1.01,7.61 v0.76,7.37 | 17.53,7.24 18.29,7.24 v18.41,7.11 | v9.33,4.95 9.33,5.02 10.16,5.84 10.16,7.62 10.54,8 12.19,8 12.57,8.38 13.97,8.38 15.11,7.24 15.49,7.24
  Top 0.203: J3.6 22.78,6.56 v22.92,6.41 | 4.7,4.95 4.57,4.95 v4.44,4.83
  Top 0.254: J3.26 22.05,12.56 22.54,12.06 v22.99,12.06 | v22.23,16.76 22.33,16.66 23.09,16.66 23.79,15.96 J3.P$1 | C8.1 4.7,4.95 | C6.1 5.23,17.8 5.59,18.16 v5.59,18.67 | J3.P$2 24.47,4.36 v24.89,3.94
  Top 0.406: BAT.- 17.78,14.48 17.14,15.11 v16.76,15.11
  Top 0.457: SIM.4 5.74,12.61 v6.48,11.87
  Route2 0.127: v2.79,17.27 2.79,16.66 2.57,16.44 arc45 2.36,15.94 2.36,15.57 2.18,15.39 2.18,14.86 2.56,14.48 | v7.3,4.83 7.37,4.83 7.64,4.55 7.72,4.55 7.77,4.5 8.99,4.5 9.4,4.9
  Bottom 0.094: U1.75 18.98,13.28 18.54,13.72 18.54,14.86 18.76,15.08 U1.72
  Bottom 0.102: U1.88 19.06,5.48 | v16.38,10.92 16.76,10.54 16.83,10.54 16.95,10.41 17.27,10.41 17.44,10.59 arc45 17.53,10.79 17.53,11.05 17.59,11.11 17.76,11.11 arc45 17.9,11.17 17.91,11.18 18.29,11.18 18.41,11.05
  Bottom 0.127: 7.55,6.68 7.62,6.6 | U1.93 16.82,4.55 17.04,4.78 | v10.29,13.08 10.67,13.08 13.46,10.29 13.46,8.64 13.97,8.13 | v11.94,13.08 11.94,12.57 13.21,11.3 13.46,11.3 13.59,11.18 | 6.29,11.87 v6.48,11.87 10.66,11.87 12.2,10.34 12.2,7.63 12.19,7.62 12.83,6.99 13.97,6.99 v14.48,6.48 | U1.5 15.92,2.88 16.06,2.73 16.06,2.29 16.05,2.29 15.9,2.13 15.9,1.42
  Bottom 0.152: U1.106 9.02,3.94 8.72,3.64 U1.17 | 11.42,4.46 U1.102 11.42,3.82 11.72,3.52 U1.12 | 19.51,5.48 U1.88 18.91,5.48 18.67,5.71 18.67,6.6 18.74,6.68 | U1.86 18.74,6.68 | 18.74,6.68 18.74,6.79 v18.41,7.11
  Bottom 0.203: U1.111 6.62,18.27 6.48,18.41 5.84,18.41 v5.59,18.67 | U1.14 10.52,3.53 10.82,3.83 U1.103 | U1.2 17.72,2.67 | U1.125 15.02,17.69 14.48,17.14 14.48,15.45 | v17.59,5.08 17.35,5.08 17.04,4.78
  Bottom 0.254: v8.25,13.08 7.11,13.08 6.98,13.21 | R19.1 11.45,0.99 v11.68,0.76 | 22.63,6.63 R13.2 20.95,6.63 | 20.95,6.63 R12.2 19.96,6.63 19.94,6.6 19.87,6.68 U1.86 | U1.123 13.82,17.76 v13.46,17.4 | R6.1 22.33,16.66 v22.23,16.76 22.15,16.69 v21.5,16.69 21.48,16.66 R5.1 | U1.55 11.72,19.59 v11.81,19.69 | U1.88 19.83,5.48 19.94,5.59 | U1.19 7.52,2.58 v7.56,2.54 | U1.17 8.72,2.81 8.45,2.54 | GSM.2 24.47,3.51 23.88,2.92 23.6,2.92 GSM.3 23.37,2.71 GSM.4 | U1.67 19.27,18.58 v19.18,18.67 | C10.1 20.95,6.63 | 22.48,15.49 23.11,15.49 23.24,15.62 23.42,15.8 24.16,15.8 24.46,15.49 24.46,14.55
  Bottom 0.305: U1.74 19.72,13.88 21.34,15.49 | U1.72 19.65,15.08 20.07,15.49
  Bottom 0.406: 21.34,15.49 22.48,15.49 22.54,15.49 v22.92,15.11 22.92,15.3 23.24,15.62
  other vias: 14.48,12.95 18.35,1.78 9.02,8.26 15.49,13.08 9.27,13.08 7.18,13.14 6.22,0.63 14.54,0.51 15.24,0.51 15.88,0.51 16.64,0.51 17.27,0.51 18.29,0.51 16.38,6.99 22.48,5.46 8.57,0.63 23.56,13.97 19.46,2.54 20.32,2.24 0.63,12.83 1.27,12.83 4.38,5.46 11.05,2.41 16.4,1.14 7.24,15.88 8.51,15.88 10.29,15.88 3.68,17.14 19.18,19.43 11.68,14.48 12.51,7.24 1.33,7.49 22.61,10.29
  pour Bottom (rank 3): 5.84,24.77 8.13,24.77 8.13,22.86 5.84,22.86
  pour GND (isolate 0.203, rank 3): 0.76,20.57 20.07,20.57 20.45,20.19 20.45,17.4 20.7,17.14 22.61,17.14 23.49,16.26 25.27,16.26 25.78,15.75 25.78,0.76 24.89,-0.13 0.63,-0.13 -0.25,0.76 -0.25,19.56
  pour Bottom (isolate 0.178, rank 3, no thermals): 0.51,20.83 19.81,20.83 20.45,20.19 20.45,17.53 20.83,17.14 22.61,17.14 23.11,16.64 23.11,16.13 26.16,13.08 26.16,0.63 25.15,-0.38 0.51,-0.38 -0.64,0.76 -0.64,19.69
  pour Route2 (isolate 0.203, rank 3): 0.51,21.21 19.56,21.21 20.45,20.32 20.45,17.65 20.83,17.27 22.48,17.27 23.11,16.64 23.11,16 26.16,12.95 26.16,0.38 25.15,-0.63 0.38,-0.63 -0.89,0.63 -0.89,19.81
  pour Top (isolate 0.203, rank 3, no thermals): 0,21.08 19.68,21.08 20.45,20.32 20.45,17.65 20.83,17.27 22.48,17.27 23.11,16.64 23.11,16 26.16,12.95 26.16,0.25 25.02,-0.89 0.38,-0.89 -1.14,0.63 -1.14,19.94
GPIO0/A0  (via drill 0.2 pad 0.46)
  Top 0.102: R25.2 7.24,4.32 7.49,4.06 9.14,4.06 9.78,4.7 9.78,5.08 10.41,5.71 11.56,5.71 12.19,6.35 v12.45,6.35
  Bottom 0.127: U1.99 13.22,5.58 v12.45,6.35
GPIO1/CTP_SCL/A1  (via drill 0.2 pad 0.46)
  Top 0.102: v18.54,2.41 18.67,2.54 18.67,4.33 19.05,4.71 19.05,4.95 19.49,5.4 20.38,5.4 20.77,5.02 22.67,5.02 23.31,5.66 J3.3
  Route2 0.102: v18.54,2.41 18.19,2.41 17.35,1.57 16.15,1.57 15.95,1.78 14.27,1.78 v14.24,1.74
  Bottom 0.102: U1.9 13.52,2.46 v14.24,1.74
GPIO2/CTP_SDA/A2  (via drill 0.2 pad 0.46)
  Top 0.102: J3.2 20.8,5.36 20.51,5.65 19.3,5.65 18.48,4.83 v18.48,4.76
  Route2 0.127: v18.48,4.76 18.41,4.7 18.41,4.32 17.02,2.92 15.37,2.92 v14.92,2.48
  Bottom 0.102: U1.8 14.12,2.9 14.54,2.48 v14.92,2.48
GPIO3/PWM1/BACKLIGHT  (via drill 0.2 pad 0.46)
  Top 0.102: J3.5 24.04,6.26 23.75,5.97 22.35,5.97 22.04,5.65 20.89,5.65 20.64,5.91 19.18,5.91 18.61,5.33 v18.22,5.33
  Route2 0.127: v12.95,2.79 14.22,2.79 14.6,3.17 16.89,3.17 18.03,4.32 18.03,5.14 v18.22,5.33
  Bottom 0.102: U1.10 12.92,2.83 v12.95,2.79
GPIO10/UART1_RX  (via drill 0.2 pad 0.46)
  Top 0.127: v16.64,16.64 17.14,16.64 17.4,16.89 17.4,17.32 17.82,17.75 18.32,17.75 18.67,17.4 18.67,17.14 19.18,16.64 20.07,16.64 20.7,16 22.73,16 23.37,15.37 23.37,14.99 23.49,14.86 23.81,14.86 24.01,14.66 J3.33
  Bottom 0.102: U1.126 15.62,17.78 16.64,16.76 v16.64,16.64
GPIO11/UART1_TX  (via drill 0.2 pad 0.46)
  Top 0.127: J3.34 20.35,14.96 19.62,15.68 18.35,15.68 v18.03,16
  Bottom 0.127: U1.127 16.22,17.82 v18.03,16
GPIO12/KCOL4  (via drill 0.2 pad 0.46)
  Top 0.102: R14.2 21.46,3.43 v21.4,3.49
  Route2 0.102: v16.51,19.81 17.65,18.67 18.16,18.67 19.05,17.78 19.05,15.49 20.19,14.35 22.14,14.35 24.13,12.36 24.13,4.95 23.37,4.19 21.97,4.19 21.4,3.62 v21.4,3.49
  Bottom 0.102: U1.63 v16.52,19.8 v16.51,19.81
GPIO13/INT2/EINT11  (via drill 0.2 pad 0.46)
  Route2 0.127: v11.18,19.69 11.18,19.3 9.27,17.4 6.73,17.4 5.33,16 3.43,16 v2.6,15.18
  Bottom 0.127: U1.54 11.12,19.63 v11.18,19.69 | R28.2 2.79,13.82 2.79,14.22 3.06,14.49 Q8.2 2.78,15 v2.6,15.18
GPIO15/KCOL1  (via drill 0.2 pad 0.46)
  Top 0.102: R9.2 24.3,3.39 23.88,3.81 23.37,3.81 22.85,4.33 v21.5,4.33
  Route2 0.102: v15.88,19.81 15.88,19.56 17.02,18.41 18.03,18.41 18.8,17.65 18.8,15.37 20.07,14.1 22.07,14.1 23.88,12.29 23.88,5.08 23.24,4.45 21.61,4.45 v21.5,4.33
  Bottom 0.102: U1.62 15.92,19.77 v15.88,19.81
GPIO17/KROW4  (via drill 0.2 pad 0.46)
  Top 0.102: R7.2 22.48,3.91 21.06,3.91 v20.97,4
  Route2 0.102: v15.24,19.81 16.89,18.16 17.78,18.16 18.54,17.4 18.54,15.24 19.94,13.84 22,13.84 23.62,12.22 23.62,5.21 23.24,4.83 21.21,4.83 20.97,4.58 v20.97,4
  Bottom 0.102: U1.61 15.32,19.73 v15.24,19.81
GPIO18/INT1/EINT13  (via drill 0.2 pad 0.46)
  Top 0.127: v12.45,16.38 12.45,16.26 11.62,15.43 6.29,15.43 5.82,14.96 R27.2 4.44,14.58 4.44,13.61 Q7.2
  Bottom 0.127: U1.118 10.82,17.76 11.05,17.53 11.43,17.53 12.45,16.51 v12.45,16.38
GPIO19/CTP_RST  (via drill 0.2 pad 0.46)
  Top 0.127: J3.31 24.17,14.06 23.69,14.54 22.73,14.54 22.48,14.8 22.48,15.34 22.07,15.75 20.57,15.75 19.94,16.38 18.92,16.38 v18.03,17.27
  Bottom 0.127: U1.128 16.82,17.85 17.14,17.53 17.78,17.53 v18.03,17.27
GPIO27/SPI_SCK  (via drill 0.2 pad 0.46)
  Top 0.102: J3.4 20.96,5.96 20.77,6.16 19.05,6.16 18.67,5.78 17.84,5.78 17.59,5.52 16.88,5.52 v16.59,5.23
  Bottom 0.102: 16.22,4.67 16.22,4.87 v16.59,5.23
  Bottom 0.127: U1.94 16.22,4.67
GPIO28/SPI_MOSI  (via drill 0.2 pad 0.46)
  Top 0.127: J3.8 20.88,7.16 20.38,6.67 17.84,6.67 v17.78,6.73
  Bottom 0.127: U1.96 15.02,4.88 16.05,5.91 17.46,5.91 17.65,6.1 17.65,6.6 v17.78,6.73
GPIO29/SPI_MISO  (via drill 0.2 pad 0.46)
  Top 0.102: J3.7 20.96,6.86 20.51,6.41 18.44,6.41 v18.24,6.21 18.25,6.22
  Bottom 0.127: U1.95 15.62,4.98 16.3,5.65 17.68,5.65 v18.24,6.21
GPIO30/EINT16
  Top 0.102: R31.1 R15.1 19.68,12.45 19.81,12.32 20.85,12.32 20.93,12.24 21.92,12.24 22.62,11.55 23.36,11.55 24.07,12.26 J3.25
GPIO38/LSRSTB  (via drill 0.2 pad 0.46)
  Top 0.102: 14.41,14.67 16.94,14.67 17.27,14.34 17.27,13.01 17.64,12.64 17.91,12.64 18.09,12.45 arc45 19.02,12.06 20.7,12.06 20.81,11.96 J3.24
  Top 0.127: 14.41,14.67 13.72,13.97 7.37,13.97 v6.86,14.48
  Bottom 0.127: U1.41 5.66,15.68 v6.86,14.48
GPIO39/LSCE_B  (via drill 0.2 pad 0.46)
  Top 0.102: J3.23 23.98,11.66 23.62,11.3 22.42,11.3 22.07,11.65 20.74,11.65 20.57,11.81 19.07,11.81 arc-45 17.84,12.32 17.53,12.32 17.02,12.83 17.02,14.22 16.89,14.35 16.64,14.35
  Top 0.127: 16.64,14.35 14.48,14.35 13.84,13.72 6.98,13.72 v6.86,13.84
  Bottom 0.127: U1.40 5.75,15.08 6.35,14.48 6.35,14.35 v6.86,13.84
GPIO43/I2C_SCL  (via drill 0.2 pad 0.46)
  Top 0.127: v3.05,11.62 3.05,11.94 3.43,12.32 4.59,12.32 4.95,12.68 4.95,14.22 5.08,14.35 6.03,14.35 6.6,14.92 13.14,14.92 v13.46,15.24 13.84,15.62 17.27,15.62 17.72,15.18 19.37,15.18 20.78,13.76 J3.30
  Bottom 0.094: U1.57 12.92,17.31 13.21,17.02
  Bottom 0.102: 13.21,17.02 13.59,16.64 13.59,15.37 v13.46,15.24
  Bottom 0.127: R22.2 2.93,10.63 Q2.2 2.93,11.5 v3.05,11.62
GPIO44/I2C_SDA  (via drill 0.2 pad 0.46)
  Top 0.127: J3.32 20.56,14.36 19.49,15.43 17.84,15.43 17.4,15.88 13.21,15.88 v13.08,15.75 | v13.08,15.75 12.83,15.49 | v2.67,8.51 2.29,8.89 2.29,9.97 2.6,10.29 2.6,12.13 3.17,12.7 4.41,12.7 4.7,12.98 4.7,14.43 4.88,14.61 5.9,14.61 6.48,15.18 12.51,15.18 v13.08,15.75
  Bottom 0.094: U1.56 12.32,17.53
  Bottom 0.127: 12.32,17.53 13.21,16.64 13.21,15.88 v13.08,15.75 | v2.67,8.51 2.93,8.25 Q1.2 2.93,7.21 R21.2
GPIO46/EAR_EINT  (via drill 0.2 pad 0.46)
  Top 0.102: v20.07,4.95 20.45,4.95 20.64,4.76 22.85,4.76 23.16,5.06 J3.1
  Bottom 0.127: R29.1 20.45,4.57 v20.07,4.95
GPIO47/LSCK0  (via drill 0.2 pad 0.46)
  Top 0.094: 20.15,10.46 22.02,10.46 22.35,10.79 23.37,10.79 23.7,10.46 J3.19
  Top 0.127: 20.15,10.46 19.94,10.67 18.03,10.67 v17.97,10.73
  Bottom 0.127: U1.42 6.24,16.28 6.48,16.51 10.92,16.51 11.18,16.26 11.18,12.95 13.97,10.16 17.4,10.16 v17.97,10.73
GPIO48/LSDA0  (via drill 0.2 pad 0.46)
  Top 0.102: J3.21 20.56,11.06 20.32,11.3 18.67,11.3 arc-37 18.29,11.43 17.72,11.43 v17.59,11.56
  Bottom 0.127: U1.44 5.89,17.48 6.35,17.02 11.18,17.02 11.68,16.51 11.68,15.62 12.95,14.35 12.95,12.32 13.33,11.94 16.51,11.94 16.95,11.49 17.53,11.49 v17.59,11.56
GPIO49/LSA0  (via drill 0.2 pad 0.46)
  Top 0.102: J3.22 20.64,11.36 20.45,11.56 18.94,11.56 arc-45 17.72,12.06 17.21,12.06 v17.14,12
  Bottom 0.127: U1.45 5.67,18.08 6.48,17.27 11.3,17.27 11.94,16.64 11.94,15.75 13.21,14.48 13.21,12.45 13.46,12.19 16.76,12.19 16.89,12.06 17.08,12.06 v17.14,12
GPIO50/LPTE  (via drill 0.2 pad 0.46)
  Top 0.094: 21.12,10.76 20.36,10.76 20.19,10.92
  Top 0.102: J3.20 21.12,10.76 | 20.19,10.92 20.07,11.05 18.41,11.05 arc45 18.11,11.18 17.91,11.18 arc45 17.9,11.17 arc-45 17.76,11.11 17.34,11.11 v17.08,10.86
  Bottom 0.127: U1.43 6.11,16.88 6.22,16.76 11.05,16.76 11.43,16.38 11.43,15.49 12.7,14.22 12.7,12.19 13.21,11.68 16.26,11.68 v17.08,10.86
INT1_H  (via drill 0.2 pad 0.46)
  Top 0.127: J1.5 1.48,10.46 v1.52,10.41 1.52,10.03 1.35,9.86 J1.7
  Top 0.305: Q7.3 1.54,14.46 J9.1
  GND 0.127: J9.1 1.29,13.7 1.9,13.08 1.9,12.57 1.27,11.94 1.27,10.67 v1.52,10.41
  Bottom 0.127: R24.2 1.8,10.69 v1.52,10.41
INT2_H  (via drill 0.2 pad 0.46)
  Top 0.127: J1.6 3.17,10.16 v2.79,9.78
  GND 0.127: v2.79,9.78 2.54,10.03 2.54,12.19 2.92,12.57 2.92,14.22 2.16,14.99 2.16,15.16 1.29,16.03 J9.2
  Bottom 0.127: Q8.3 3.41,16.24 3.41,16.4 | R26.2 2.67,9.91 v2.79,9.78
  Bottom 0.305: Q8.3 3.16,16.64 1.42,16.64 J9.2
MICBIAS0  (via drill 0.2 pad 0.46)
  Top 0.102: J3.14 20.76,8.96 20.64,9.08 15.68,9.08
  Top 0.127: 15.68,9.08 14.48,10.29 11.49,10.29 v11.37,10.16
  Bottom 0.127: U1.30 5.77,9.08 6.6,9.91 11.11,9.91 v11.37,10.16
N$1  (via drill 0.2 pad 0.46)
  Top 0.102: R15.2 18.75,12.45 arc-45 18.28,12.64 17.84,13.08 v17.78,13.08
  Bottom 0.127: v17.78,13.08 17.65,12.95 17.65,12.57 17.53,12.45 13.72,12.45 13.46,12.7 13.46,14.61 12.64,15.43 12.64,15.94 12.95,16.26 12.95,16.51 12.02,17.45 U1.120
N$2  (via drill 0.2 pad 0.46)
  Route2 0.102: v20.22,2.82 20.04,2.82 19.86,3 18.24,3 17.68,2.44 16.15,2.44 15.75,2.03 14.76,2.03 14.38,2.41 11.91,2.41 11.53,2.79 10.67,2.79 v10.29,2.41
  Bottom 0.094: U1.104 10.22,2.6
  Bottom 0.102: 10.23,2.6 10.22,2.6 10.22,2.48 v10.29,2.41 | R29.2 20.45,3.05 v20.22,2.82
N$3
  Bottom 0.102: U1.98 13.82,2.75 14.64,1.93 R30.1
N$4
  Bottom 0.127: R3.2 22.71,16.13 R6.2 22.76,16.13 22.89,16.13 arc45 23.49,16.38 23.55,16.43 BT.1
N$5
  Bottom 0.102: R12.1 | 21.03,6.07 R8.1
  Bottom 0.127: U1.87 R12.1 | R12.1 21.03,6.07
N$6  (via drill 0.2 pad 0.46)
  Top 0.127: R31.2 18.61,12.95 v18.41,13.14
  Bottom 0.127: v18.41,13.14 17.91,13.65 17.91,15.24 18.54,15.88 18.54,17.53 18.02,18.05 U1.130
N$7
  Bottom 0.102: 21.64,6.07 R8.2 | R13.1 22.25,6.07
  Bottom 0.127: R13.1 21.64,6.07 | GSM.1 23.37,5.21 22.68,5.89 arc45 22.25,6.07
N$8  (via drill 0.2 pad 0.46)
  Top 0.102: PWR.1 9.68,2.06 9.27,1.65 6.86,1.65 v6.73,1.78
  Bottom 0.102: R1.1 C11.2 6.7,0.99 D3.1 6.35,1.4 v6.73,1.78
N$9
  Bottom 0.127: U1.73 19.36,14.48 arc45 19.91,14.7 20.49,15.28 arc45 20.57,15.49 arc-45 R5.2 21.54,16.1 R3.1
N$10
  Bottom 0.127: R1.2 8.15,1.55 8.76,2.16 9.27,2.16 9.92,2.81 U1.15
N$12
  Top 0.254: C8.2 R17.2 R25.1 R23.1
N$18  (via drill 0.2 pad 0.46)
  Top 0.127: R32.2 20.8,16.89 19.3,16.89 18.99,17.21 18.99,17.59 17.14,19.43 v17.14,19.81
  Bottom 0.127: U1.64 17.12,19.79 v17.14,19.81
N$20
  Bottom 0.102: U1.101 12.02,2.69
  Bottom 0.127: R20.2 9.88,1.55 | R10.2 8.91,1.55 9.02,1.65 9.8,1.65 R20.2 | R20.2 10.26,1.9 11.23,1.9 12.02,2.69
N$21
  Bottom 0.102: R19.2 11.3,1.55 12.32,2.57
  Bottom 0.127: U1.11 12.32,2.57 | R11.2 R19.2
N$32
  Top 0.102: LED.1 24.49,2.62 23.69,3.43 R7.1
N$33
  Top 0.102: LED.2 24.49,1.12 24.67,1.3 arc45 25.02,2.15 25.02,3.2 R9.1
N$34
  Top 0.102: LED.4 23.64,1.44 23.21,1.88 arc-45 23.11,2.1 23.11,2.69 R14.1
RESETB  (via drill 0.2 pad 0.46)
  Top 0.127: R2.1 C17.2 3.02,16.23 v2.86,16.07 2.9,16.1
  Route2 0.127: v10.54,19.69 10.54,19.3 9.14,17.91 6.6,17.91 4.95,16.26 3.05,16.26 v2.86,16.07
  Bottom 0.127: U1.53 10.52,19.66 v10.54,19.69
SCL_H  (via drill 0.2 pad 0.46)
  Top 0.127: J1.3 1.43,11.06 1.78,11.41 v1.78,11.56 2.16,11.18 2.16,10.29 1.13,9.26 J1.9
  GND 0.127: J10.2 1.52,3.81 2.5,4.79 2.5,7.79 2.16,8.13 2.16,11.18 v1.78,11.56
  Bottom 0.127: Q2.3 2.78,12.3 2.03,11.56 v1.78,11.56 1.8,11.58 R18.2
SDA_H  (via drill 0.2 pad 0.46)
  Top 0.127: v2.79,9.14 3.21,9.56 J1.8 4.23,9.56 4.44,9.78 4.44,10.51 4.19,10.76 J1.4
  GND 0.127: J10.1 1.29,2.05 2.83,3.59 2.83,7.91 3.17,8.26 3.17,8.76 v2.79,9.14
  Bottom 0.127: 3.19,9 Q1.3 2.94,9 v2.79,9.14 2.67,9.27 R16.2
SIM2_SCLK/GPIO42  (via drill 0.2 pad 0.46)
  Top 0.127: SIM.3 12.47,18.56 10.79,16.89 5.31,16.89 C3.2 4.8,16.94 arc-45 4.72,17.13 4.72,17.79 arc-45 4.87,18.14 5.08,18.35 v5.08,19.56
  Route2 0.127: v9.27,19.69 9.27,19.56 8.89,19.18 6.6,19.18 6.08,19.7 5.22,19.7 v5.08,19.56
  Bottom 0.127: U1.51 9.32,19.64 v9.27,19.69
SIM2_SIO/GPIO40  (via drill 0.2 pad 0.46)
  Top 0.127: SIM.7 13.02,6.66 12.89,6.79 12,6.79 v11.94,6.86 | v4.32,6.73 4.85,7.26 C7.2
  GND 0.127: v8.64,19.69 7.37,19.69 5.84,18.16 5.46,18.16 3.43,16.13 3.43,12.83 3.68,12.57 3.68,7.37 v4.32,6.73 4.44,6.6 6.98,6.6 7.49,7.11 10.79,7.11 10.92,6.99 11.81,6.99 v11.94,6.86
  Bottom 0.127: U1.50 8.72,19.6 v8.64,19.69
SIM2_SRST/GPIO41/CLKO3  (via drill 0.2 pad 0.46)
  Top 0.127: SIM.2 10.97,17.95 10.16,17.14 5.24,17.14 C6.2 5.18,17.25 6.1,18.16 6.1,18.92 v5.71,19.3
  Bottom 0.127: U1.49 8.12,19.44 7.86,19.69 5.98,19.69 5.71,19.43 v5.71,19.3
SPK_OUTN  (via drill 0.2 pad 0.46)
  Top 0.102: J3.9 20.35,7.46 20.19,7.62 19.75,7.62
  Top 0.152: v8.64,4.95 9.08,5.4 9.33,5.4 9.78,5.84 9.78,7.75 10.35,8.32 12.06,8.32 12.43,8.69 14.05,8.69 15.11,7.62 19.75,7.62
  Bottom 0.152: U1.107 8.42,4.74 v8.64,4.95
SPK_OUTP  (via drill 0.2 pad 0.46)
  Top 0.152: v8,4.95 8.76,5.71 9.14,5.71 9.4,5.97 9.4,7.87 10.16,8.64 11.94,8.64 12.32,9.02 14.16,9.02 15.24,7.94 20.26,7.94 20.43,7.76 J3.10
  Bottom 0.102: U1.18 8.12,4.83 v8,4.95
USB_5V  (via drill 0.3 pad 0.61)
  Top 0.305: 11.07,4.28 C4.2 | C98.1 10.25,4.28 | USB.1 15.08,4.35
  Bottom 0.305: U1.25 6.12,6.08 6.48,5.71
  Bottom 0.61: 6.48,5.71 9.52,5.71
  Bottom 0.635: 9.52,5.71 9.91,5.71 v10.54,5.08
  pour Top (no thermals): 10.54,5.46 11.94,5.46 12.32,5.84 14.22,5.84 15.24,4.83 15.24,3.56 15.11,3.43 14.6,3.43 14.22,3.81 14.22,4.32 13.72,4.83 12.45,4.83 11.68,4.06 10.79,4.06 10.67,4.19 10.16,4.19 10.03,4.32 10.03,4.95
USB_DM  (via drill 0.2 pad 0.46)
  Top 0.127: v12.7,7.87 13.08,7.49 14.1,7.49 15.56,6.03 D14.1 15.73,5.8 USB.2
  Bottom 0.127: U1.36 5.69,12.68 5.84,12.83 6.35,12.83 7.05,12.13 10.88,12.13 12.7,10.31 v12.7,7.87
USB_DP  (via drill 0.2 pad 0.46)
  Top 0.127: USB.3 16.38,4.7 16,5.08 16,5.53 D6.1 16.44,6.17 16,6.6 15.37,6.6 14.22,7.75 13.53,7.75 v13.33,7.94
  Bottom 0.127: U1.37 6.28,13.28 7.18,12.38 10.99,12.38 12.95,10.41 12.95,8.32 v13.33,7.94
VBAT  (via drill 0.2 pad 0.46, 0.25 pad 0.51)
  Top 0.254: 20.75,13.16 J3.28 22.08,13.16 v22.23,13.02 22.38,12.86 J3.27 | 4,8.96 4.13,8.96 4.83,9.65 4.83,10.79 4.26,11.36 J1.2 | R17.1 5.31,3.83 v5.46,3.68 | R4.1 15.39,18.82 13.97,17.4 v13.97,16.89
  Top 0.305: 4,8.96 J1.10 | J1.10 3.63,8.96 | 3.43,8.64 3.49,8.64 J1.10
  Top 0.61: 3.43,8.64 3.43,8 1.54,6.11 J10.3
  GND 0.305: 20.07,12.45 17.65,12.45 13.97,16.13 v13.97,16.89 | v17.02,1.97 17.02,2.03 16.64,2.41 16.38,2.16 v16.38,1.97
  GND 0.762: 16.64,2.41 16.64,3.43 15.88,4.19
  Bottom 0.152: C15.2 22.16,13.53
  Bottom 0.203: U1.59 14.12,18.77 14.42,18.47 U1.124 | U1.110 6.62,4.21
  Bottom 0.254: 14.42,17.85 14.42,17.72 13.97,17.27 v13.97,16.89
  Bottom 0.305: U1.124 14.42,17.85 | C5.2 17.25,1.74 v17.02,1.97 17.12,2.07 U1.3 | U1.4 16.52,2.1 v16.38,1.97
  other vias: 4.7,4.06 20.32,12.76 20.32,13.34
  pour Bottom (isolate 0.203, no thermals): 0.76,6.86 1.52,6.86 3.17,5.21 3.17,4.7 3.43,4.45 6.48,4.45 6.73,4.19 6.73,4.06 6.6,3.94 6.22,3.94 5.46,3.17 3.3,3.17 2.41,4.06 2.41,4.32 1.65,5.08 0.76,5.08 0.38,5.46 0.38,6.48
  pour Bottom (isolate 0.203, no thermals): 21.46,14.99 22.23,14.99 22.48,14.73 22.48,13.08 22.61,12.95 22.61,11.68 21.84,10.92 21.84,8.38 21.59,8.13 20.19,8.13 20.19,12.06 19.94,12.32 19.94,13.46
  pour GND (isolate 0.203): 4.83,3.3 5.97,3.3 6.35,3.68 6.35,4.32 7.49,5.46 10.79,5.46 12.83,3.43 16.13,3.43 16.64,3.94 16.64,5.97 22.61,11.94 22.61,12.95 21.97,13.59 19.94,13.59 19.68,13.34 19.68,11.56 15.24,7.11 14.86,7.11 13.59,5.84 12.45,5.84 11.3,6.99 6.35,6.99 4.44,4.95 4.44,3.68
  pour Top (isolate 0.203, no thermals): 18.8,14.86 19.18,14.86 20.7,13.34 20.7,12.7 20.45,12.45 19.94,12.45 19.68,12.7 19.68,13.08 19.3,13.46 18.8,13.46 18.54,13.72 18.54,14.61
VIO28_LDO  (via drill 0.2 pad 0.46)
  Top 0.203: LED.3 23.64,2.01 23.7,2.01 v23.94,1.78
  Top 0.254: v18.03,16.64 18.16,16.64 18.8,16 19.81,16 20.45,15.37 21.97,15.37 22.16,15.18 22.16,13.88 22.59,13.46 v24,13.46 | v4.32,15.49 4.34,15.52 R27.1 4.85,15.54 | 4.29,15.47 v4.32,15.49 | v2.41,13.34 2.52,13.22 Q7.1 3.68,13.84 3.94,13.84 4.06,13.97 4.06,15.24 v4.32,15.49 | R2.2 4.04,15.21 v4.32,15.49
  Top 0.305: J3.29 v24,13.46 | C12.2 3.94,15.88 v4.32,15.49
  Route2 0.203: v23.94,1.78 23.88,1.84 23.88,3.68 24.77,4.57 24.77,12.7 v24,13.46
  Route2 0.254: v18.03,16.64 17.65,16.64 15.49,18.8 14.6,18.8 13.72,19.69 v13.72,19.81
  Route2 0.305: v13.72,19.81 12.83,19.81 9.91,16.89 6.86,16.89 5.46,15.49 v4.32,15.49
  GND 0.254: v3.68,6.6 3.3,6.22 3.3,4.02 6.18,1.14 v9.4,1.14 9.7,1.14 10.39,1.83 11.28,1.83 12.75,3.3 13.41,3.3 14.73,1.98 14.73,1.46 14.33,1.07 v14.22,1.07
  Bottom 0.254: R11.1 R20.1 9.55,0.99 v9.4,1.14 | v4.32,15.49 4.06,15.23 Q8.1 3.3,14.25 R28.1 | Q2.1 | Q2.1 3.93,11.61 4,11.68 4,12.69 3.8,12.89 2.92,12.89 2.48,13.34 v2.41,13.34 | TP2.T 4.19,9.93 R22.1 3.93,10.38 Q2.1 | R21.1 3.71,6.63 v3.68,6.6 | v14.22,1.07 14.63,1.07 R34.2
  Bottom 0.305: U1.58 13.52,19.62 v13.72,19.81 | R21.1 3.71,7.54 Q1.1 3.93,8.25 4.06,8.38 4.06,9.53 TP2.T
VIO33_LDO  (via drill 0.2 pad 0.46)
  Route2 0.254: v4.06,6.1 5.08,6.1 7.11,4.06 12.57,4.06 13.33,3.3 14.22,3.3 14.48,3.56 16.57,3.56 17.08,4.07 17.08,6.79 17.91,7.62 19.56,7.62 v20,7.18
  Bottom 0.254: R18.1 R24.1 1.02,10.76 1.02,10.13 R26.1 R16.1 1.24,9.04 1.84,8.45 | v4.06,6.1 3.36,6.1 2.29,7.17 2.29,8 1.84,8.45 | 24.13,6.73 TP5.T 23.41,7.45 U2.2 23.37,7.52 C10.2 20.34,7.52 v20,7.18 | C13.2 1.84,8.45
VRTC  (via drill 0.2 pad 0.46)
  Top 0.102: 14.73,19.56 v14.48,19.81
  Top 0.127: R4.2 14.83,19.46 v14.48,19.81
  Bottom 0.102: U1.60 14.72,19.57 v14.48,19.81
VSIM2  (via drill 0.2 pad 0.46, 0.25 pad 0.51)
  Top 0.254: SIM.1 9.36,18.56 9.93,19.14 v9.93,19.69 | SIM.6 10.97,7.16 v11.3,7.49 | v6.86,7.18 6.73,7.05 6.73,6.6 6.25,6.12 C14.1 C2.1
  GND 0.254: v9.93,19.69 9.93,19.46 9.52,19.05 7.24,19.05 5.97,17.78 5.71,17.78 3.81,15.88 3.81,14.61 4.06,14.35 4.06,7.49 4.32,7.24 4.7,7.24 4.95,6.99 6.67,6.99 v6.86,7.18 7.18,7.49 v11.3,7.49
  Bottom 0.254: U1.52 9.92,19.67 v9.93,19.69

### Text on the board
tPlace: 6 | 5 | 4 | + | - | 3 | GSM+BLE | 2 | V1.0 | 1
bPlace: 6 | 5 | 4 | 3 | 2 | 1
dxf: B | B | B | B | B
tDocu: P3
Enhance: Enhance Area, / Torence +/-0.03mm, / Total Thickness = 0.2mm

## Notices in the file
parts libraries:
moudle-new: This work is licensed under the Creative Commons Attribution 4.0 International License.
To view a copy of this license,visit:
http://creativecommons.org/licenses/by-sa/4.0
moudle-new: CC-BY-SA
